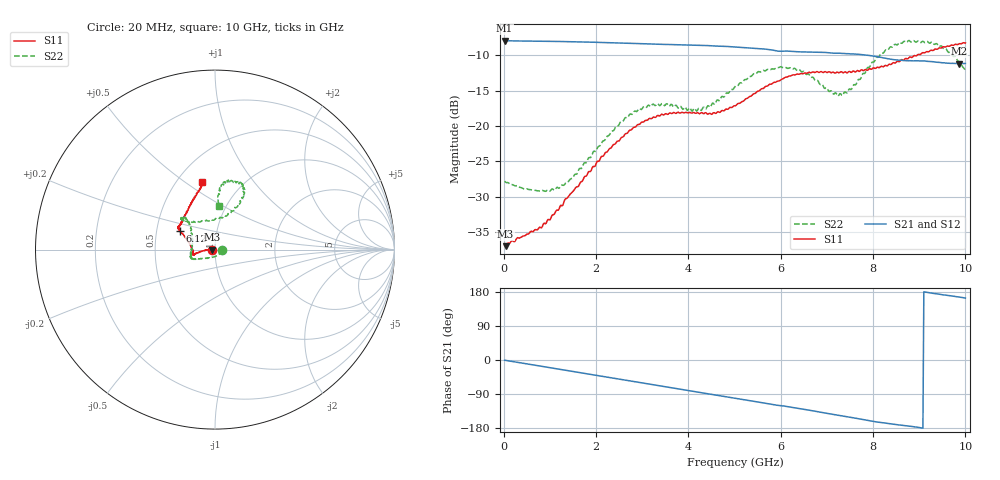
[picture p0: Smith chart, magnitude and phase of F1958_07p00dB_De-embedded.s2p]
! Integrated Device Technology
! Corporate Headquarters
! 6024 Silver Creek Valley Road
! San Jose, CA 95138  USA
! Phone:  1-408-284-8200
! Toll Free:  1-800-223-1366
! Webpage:  http://www.idt.com/
! Timing and RF Division
! 515 Groton Road, Suite 102
! Westford, MA 01886-6024
! Device:  F1958
! Description: 7-bit 0.25 dB Digital Step Attenuator
! Frequency:  0.001 -  6.000 GHz
! Package:  4x4 mm Thin QFN Plastic Package: 24 pin
! Ports:  2 RF, 12 DC
!  Pin  1  = D0
!  Pin  2  = VDD
!  Pin  3  = VMODE
!  Pin  4  = GND
!  Pin  5  = RF1  =  Port 1
!  Pin  6  = GND
!  Pin  7  = GND
!  Pin  8  = GND
!  Pin  9  = GND
!  Pin 10  = GND
!  Pin 11  = GND
!  Pin 12  = GND
!  Pin 13  = GND
!  Pin 14  = RF2  =  Port 2
!  Pin 15  = GND
!  Pin 16  = LE
!  Pin 17  = CLK
!  Pin 18  = DATA
!  Pin 19  = D6
!  Pin 20  = D5
!  Pin 21  = D4
!  Pin 22  = D3
!  Pin 23  = D2
!  Pin 24  = D1
! State:  28
! Atten State:  7.00 dB
! Voltage:  +3.30 Volts
! Current:  0.257 mA
! Data:  The device was measured on a F1958 evaluation board which has
!  individual transmission lines to the RF pins.  Data was collected
!  using a calibrated network analyzer.  The evaluation board was
!  de-embedded using Automatic Fixture Removal (AFR).
!  The reference plane is the edge of the package pin.
! Misc:
!  Action Tracker AT0419
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# GHz S dB R 50
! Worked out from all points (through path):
!   500 points, 20 MHz to 10 GHz, reference 50 ohm
!   highest |S21| = -7.96 dB at 20 MHz (marker M1); lowest = -11.2 dB at 9.86 GHz (marker M2)
!   group delay of S21, straight-line fit = 55.2 ps
!   lowest |S11| = -36.9 dB at 40 MHz (marker M3), VSWR 1.03, Z = 48.6 - j0.0879 ohm
!   |S11| at or under -10 dB: start of sweep to 8.958 GHz
!   |S22| runs from -29.2 to -7.9 dB; largest |S21 - S12| = 0.0011
!   S11 on the Smith chart (normalised r, x): 20 MHz: 0.97, -0.00; 6.12 GHz: 0.66, +0.14; 10 GHz: 0.66, +0.59
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0.02  -36.87 -176.8  -7.96 -0.6  -7.96 -0.5  -27.78 -3.7
0.04  -36.95 -176.4  -7.97 -1.0  -7.97 -0.9  -27.93 -5.6
0.98  -33.20 178.8  -8.06 -19.8  -8.06 -19.8  -29.14 -60.9
1.34  -30.27 -178.3  -8.11 -27.1  -8.10 -27.1  -28.04 -93.1
1.7  -27.81 -176.5  -8.16 -34.2  -8.15 -34.2  -25.86 -119.7
2.62  -21.23 -171.0  -8.32 -52.7  -8.31 -52.7  -18.93 -152.5
2.96  -19.66 -169.2  -8.39 -59.5  -8.38 -59.6  -17.62 -155.7
3.36  -18.57 -166.7  -8.48 -67.5  -8.48 -67.6  -17.01 -160.7
4.3  -18.14 -170.8  -8.64 -86.3  -8.66 -86.4  -17.61 164.1
5.02  -17.15 170.1  -8.85 -101.0  -8.86 -101.0  -14.39 136.9
5.54  -15.03 158.0  -9.10 -111.5  -9.11 -111.5  -12.37 133.7
6.12  -13.12 152.6  -9.44 -122.6  -9.46 -122.6  -11.78 137.2
6.68  -12.42 148.7  -9.59 -133.7  -9.60 -133.6  -13.12 133.5
7.1  -12.49 145.2  -9.70 -142.8  -9.71 -142.7  -15.06 114.5
7.34  -12.48 144.0  -9.77 -147.8  -9.78 -147.6  -15.71 92.7
7.58  -12.25 140.4  -9.85 -152.6  -9.85 -152.5  -14.18 74.9
7.9  -12.03 133.0  -10.04 -159.7  -10.03 -159.8  -11.73 65.0
8.34  -11.33 123.3  -10.54 -168.1  -10.54 -168.2  -9.15 62.2
8.76  -10.50 114.0  -10.81 -174.2  -10.81 -174.2  -8.00 68.1
9.26  -9.33 105.7  -10.93 176.6  -10.93 176.6  -8.19 79.5
9.86  -8.43 100.5  -11.21 166.2  -11.24 166.3  -10.91 85.6
10  -8.30 100.6  -11.19 163.3  -11.22 163.4  -12.16 84.7
